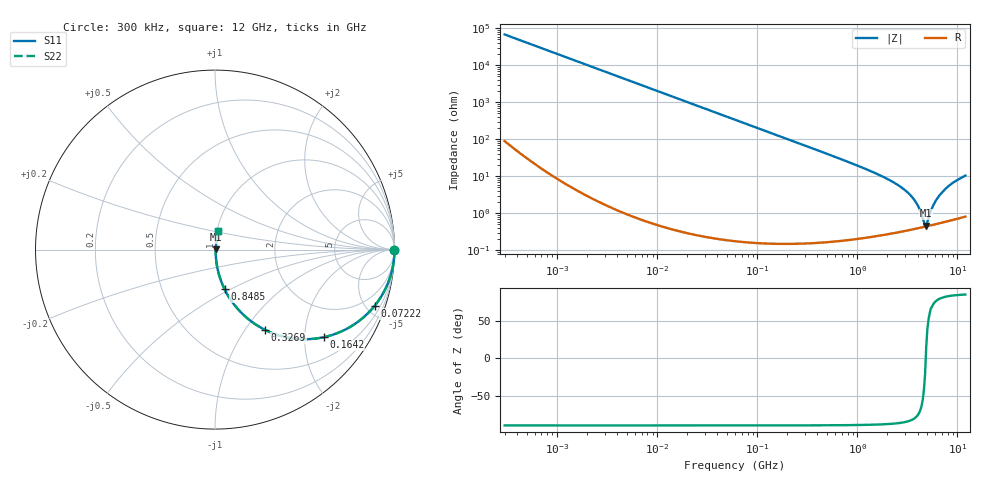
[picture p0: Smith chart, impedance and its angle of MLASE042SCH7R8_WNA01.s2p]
! MLASE042SCH7R8_WNA01  S-PARAMETER MODEL  ( General Type )
! Model Generated by TAIYO YUDEN Corporation (http://www.ty-top.com)
! Version 1.0
! TAIYO YUDEN Control No. 120810
! Copyright(c) 2012 TAIYO YUDEN CO.,LTD. All Rights Reserved.
! Product Description (link to TY-COMPAS)
! https://ds.yuden.co.jp/TYCOMPAS/or/detail?pn=MLASE042SCH7R8BWNA01&u=M
! Products Name : Multilayer Ceramic Capacitors
! Characteristics :
!  Capacitance : 7.8 pF , Rated Voltage : 16V , TCC : CH / C0H
!  Case Size : 0.4 x 0.2 / 0.016 x 0.008 [mm/inch] , Thickness : 0.2 / 0.008 [mm/inch]
!  (Conditions: Temperature = 25 degC , DC Bias Current/Voltage = 0A / 0V)
! External Node Assignments :
!  1  o---| |---o  2
! GND o---------o GND
! Frequency Range : 0.3MHz  -  12000MHz  [ 401 STEP ]
# MHz S RI R 50
! Freq[MHz].  S11 Real  S11 Imag  S21 Real  S21 Imag  S12 Real  S12 Imag  S22 Real  S22 Imag
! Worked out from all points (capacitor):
!   401 points, 300 kHz to 12 GHz, reference 50 ohm
!   read as one part in series: C = 7.79 pF near 316.3 kHz
!   lowest |Z| = 460 mohm at 4.875 GHz (marker M1)
!   series resonance near 4.823 GHz, so ESL is about 140 pH
!   S11 on the Smith chart (normalised r, x): 300 kHz: open; 72.22 MHz: 1.00, -5.66; 164.2 MHz: 1.00, -2.49; 326.9 MHz: 1.00, -1.24; 848.5 MHz: 1.00, -0.47; 12 GHz: 1.02, +0.21
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0.3  1 -0.00147  4.08e-06 0.00147  4.08e-06 0.00147  1 -0.00147
1.769972  0.9999 -0.00866  7.77e-05 0.00866  7.77e-05 0.00866  0.9999 -0.00866
10.44266  0.9974 -0.051  0.00262 0.051  0.00262 0.051  0.9974 -0.051
27.10171  0.9827 -0.1304  0.0173 0.1304  0.0173 0.1304  0.9827 -0.1304
60  0.9204 -0.2704  0.0796 0.2704  0.0796 0.2704  0.9204 -0.2704
72.22496  0.8887 -0.3142  0.1113 0.3142  0.1113 0.3142  0.8887 -0.3142
164.1901  0.6068 -0.4879  0.3932 0.4879  0.3932 0.4879  0.6068 -0.4879
326.9496  0.2794 -0.4475  0.7206 0.4475  0.7206 0.4475  0.2794 -0.4475
353.9943  0.2484 -0.4307  0.7516 0.4307  0.7516 0.4307  0.2484 -0.4307
526.7124  0.1291 -0.3332  0.8709 0.3332  0.8709 0.3332  0.1291 -0.3332
848.5281  0.0533 -0.2205  0.9467 0.2205  0.9467 0.2205  0.0533 -0.2205
2088.533  0.00901 -0.0787  0.991 0.0787  0.991 0.0787  0.00901 -0.0787
2795.104  0.00555 -0.0483  0.9944 0.0483  0.9944 0.0483  0.00555 -0.0483
3454.93  0.00444 -0.0288  0.9956 0.0288  0.9956 0.0288  0.00444 -0.0288
4050.141  0.00418 -0.015  0.9958 0.015  0.9958 0.015  0.00418 -0.015
4623.766  0.00429 -0.00385  0.9957 0.00385  0.9957 0.00385  0.00429 -0.00385
4875.354  0.00442 0.00121  0.9956 -0.00121  0.9956 -0.00121  0.00442 0.00121
5006.236  0.0045 0.00369  0.9955 -0.00369  0.9955 -0.00369  0.0045 0.00369
5715.274  0.00512 0.0153  0.9949 -0.0153  0.9949 -0.0153  0.00512 0.0153
6879.757  0.00666 0.034  0.9933 -0.034  0.9933 -0.034  0.00666 0.034
8732.115  0.0103 0.0618  0.9897 -0.0618  0.9897 -0.0618  0.0103 0.0618
12000  0.0187 0.1019  0.9813 -0.1019  0.9813 -0.1019  0.0187 0.1019
